VAR_GLOBAL CONSTANT
	// Streaming
	cOversamples 		: UDINT 	:= 10;									// number of oversamples
	cBufferLength		: UDINT		:= 400;									// buffer size
	
	// Parameters for RainflowCounting and MinersRule
	cRfRangeBins 		: UDINT 	:= 100;									// Number of stress range bins
	cRfMeanBins			: UDINT		:= 100;									// Number of mean stress bins
	cStressMin			: LREAL		:= -50.0;								// Minimum negative stress [here in MPa]
	cStressMax			: LREAL		:= +50.0;								// Maximum positive stress [here in MPa]
	
	// Configuration for Range-Mean counting
	cRfRangeMin			: LREAL		:= 0;									// less or equal min modulated amplitude of signal
	cRfRangeMax			: LREAL		:= cStressMax - cStressMin;			 	// greater or equal max modulated amplitude of signal
	cRfMeanMin			: LREAL		:= cStressMin; 							// lower limit of mean stress
	cRfMeanMax			: LREAL		:= cStressMax;							// upper limit of mean stress

	// Numerical range and mean stress resolution
	cBinWidthRange		: LREAL		:= (cRfRangeMax - cRfRangeMin) / cRfRangeBins;	     // Width of stress bins
	cBinWidthMean		: LREAL		:= (cRfMeanMax - cRfMeanMin) / cRfMeanBins;	         // Width of mean stress bins
	
	// Mean stress correction
	// Load cycle correction to account for mean stress effects
	cMSCType 			: E_CM_MeanStressCorrection := E_CM_MeanStressCorrection.eCM_Goodman; //  also no or Gerber correction avaiable
	
	// Material definition; Woehler curve [here defined in MPa according to input signal]
	// Following parameters need to be set according to used material
	cSRI				: LREAL		:= 350;    // Stress Range Intercept (extrapolated Woehler curve to N = 1 with gradient cK1)
	// Hint: SRI is larger than UTS from material definition point of view. However, this is adopted in this sample to get faster reaction.
    cUTS				: LREAL		:= 700;    //  Ultimate Tensile Strength of the material (max. limit until failure occurs). 
	cUseUTSCorrection	: BOOL 		:= TRUE;  
	cK1					: LREAL		:= 3;      // Gradient of Woehler Curve for region N = 1 to cNc1  
	cK2					: LREAL		:= 5;      // Gradient of Woehler Curve starting from cNC2  
	cNC2 				: ULINT		:= 100000; // Fatigue Transition Point between cK1 and cK2
	cNC1				: ULINT		:= 100;    // Transition Point for UTS correction (limits Woehler curve to UTS as max. value)  	
	cRRatio				: LREAL		:= -1.0;   // R-Ratio of the material test (-1 defines a test with fully-reversed cyclic load) 
	
	// user defined, see MAIN_CM.configure first few commented code lines
	// cCyclesToFailure	: LREAL		:= 1000;		// Number of stress cycles until predicted end of lifetime.
	
	// Base damage from previous runs; to be managed by user.
	cBaseDamage			: LREAL		:= 0.0;
	nBaseCycles			: ULINT		:= 0;
END_VAR
